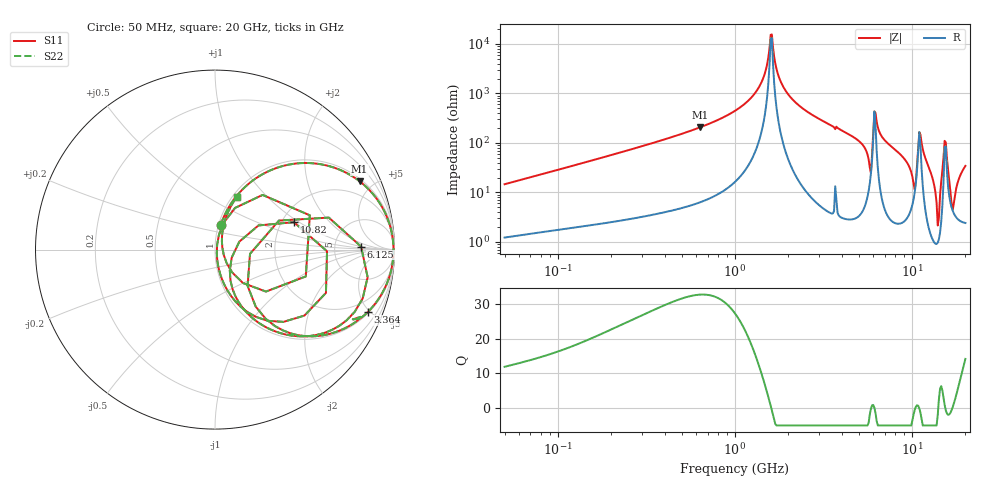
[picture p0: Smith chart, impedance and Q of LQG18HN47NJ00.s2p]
!Murata Part Number: LQG18HN47NJ00
!These Parameters are Measured in Series Mode Connection
!  o--[Z]--o
!Port1  Port2
!  o-------o
!Freq. Start=50[MHz] Stop=20[GHz], 401[Steps]
# Hz S RI R 50
!Freq.(Hz) S11(Real) S11(Imag) S21(Real) S21(Imag) S12(Real) S12(Imag) S22(Real) S22(Imag)
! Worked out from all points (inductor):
!   401 points, 50 MHz to 20 GHz, reference 50 ohm
!   read as one part in series: L = 46.1 nH near 51.52 MHz
!   highest Q = 32.7 at 638 MHz (marker M1), where L = 51.9 nH
!   self-resonance near 1.591 GHz
!   S11 on the Smith chart (normalised r, x): 50 MHz: 1.02, +0.29; 3.364 GHz: 1.08, -4.86; 6.125 GHz: 9.65, +0.97; 10.82 GHz: 2.32, +0.91; 20 GHz: 1.05, +0.69
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5e7  0.0323 0.1397  0.9677 -0.1397  0.9677 -0.1397  0.0323 0.1397
1.364002e8  0.1442 0.3258  0.8558 -0.3258  0.8558 -0.3258  0.1442 0.3258
3.721004e8  0.5418 0.4813  0.4582 -0.4813  0.4582 -0.4813  0.5418 0.4813
6.380365e8  0.8055 0.3808  0.1945 -0.3808  0.1945 -0.3808  0.8055 0.3808
1e9  0.9452 0.21  0.0548 -0.21  0.0548 -0.21  0.9452 0.21
1.369645e9  0.9888 0.0717  0.0112 -0.0717  0.0112 -0.0717  0.9888 0.0717
1.614971e9  0.9946 -0.00338  0.00542 0.00338  0.00542 0.00338  0.9946 -0.00338
1.904239e9  0.9885 -0.0797  0.0115 0.0797  0.0115 0.0797  0.9885 -0.0797
2.728004e9  0.9275 -0.2493  0.0725 0.2493  0.0725 0.2493  0.9275 -0.2493
3.364474e9  0.8511 -0.3478  0.1489 0.3478  0.1489 0.3478  0.8511 -0.3478
5.117541e9  0.5092 -0.4825  0.4908 0.4825  0.4908 0.4825  0.5092 -0.4825
5.683258e9  0.2268 -0.3175  0.7732 0.3175  0.7732 0.3175  0.2268 -0.3175
6.125241e9  0.8138 0.0169  0.1862 -0.0169  0.1862 -0.0169  0.8138 0.0169
6.601595e9  0.6912 -0.4255  0.3088 0.4255  0.3088 0.4255  0.6912 -0.4255
7.442007e9  0.4594 -0.4824  0.5406 0.4824  0.5406 0.4824  0.4594 -0.4824
1.019291e10  0.0824 -0.1158  0.9176 0.1158  0.9176 0.1158  0.0824 -0.1158
1.082228e10  0.4398 0.1528  0.5602 -0.1528  0.5602 -0.1528  0.4398 0.1528
1.166392e10  0.2927 -0.3966  0.7073 0.3966  0.7073 0.3966  0.2927 -0.3966
1.396067e10  0.00993 -0.0189  0.9901 0.0189  0.9901 0.0189  0.00993 -0.0189
1.527346e10  0.5283 0.191  0.4717 -0.191  0.4717 -0.191  0.5283 0.191
1.696185e10  0.041 0.0107  0.959 -0.0107  0.959 -0.0107  0.041 0.0107
2e10  0.122 0.2939  0.878 -0.2939  0.878 -0.2939  0.122 0.2939
